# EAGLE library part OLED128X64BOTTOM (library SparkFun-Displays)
Micro OLED TODO: Add description SparkFun Products: product
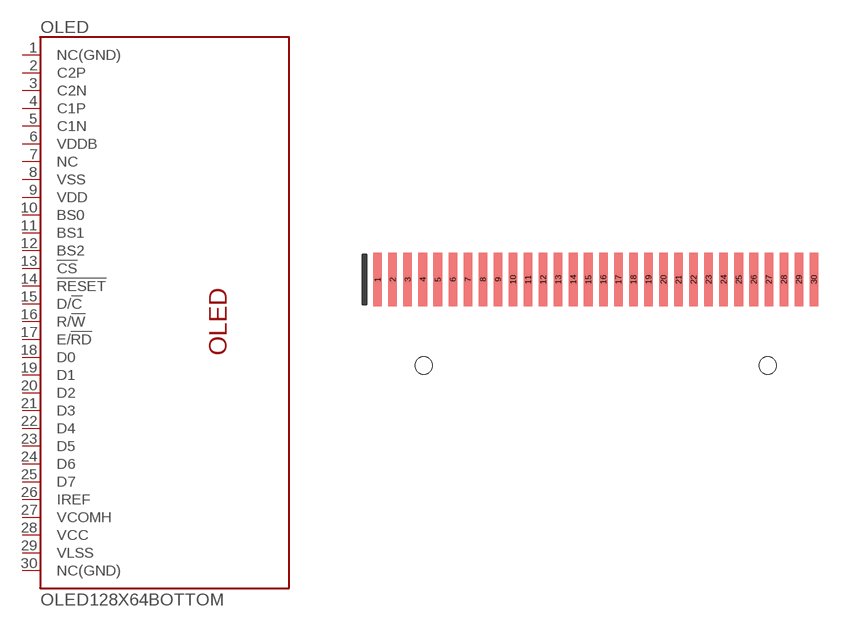
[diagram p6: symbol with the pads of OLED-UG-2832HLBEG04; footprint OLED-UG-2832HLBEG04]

Designator prefix OLED

## OLED128X64BOTTOM  [OLED-UG-2832HLBEG04]
1  NC(GND)
2  C2P
3  C2N
4  C1P
5  C1N
6  VDDB
7  NC
8  VSS
9  VDD
10  BS0
11  BS1
12  BS2
13  !CS!
14  !RESET!
15  D/!C!
16  R/!W!
17  E/!RD!
18  D0
19  D1
20  D2
21  D3
22  D4
23  D5
24  D6
25  D7
26  IREF
27  VCOMH
28  VCC
29  VLSS
30  NC(GND)

## Footprint OLED-UG-2832HLBEG04 (pad centres in mm)
OLDE display Specifications: Pin count: 30 Pin pitch: 0.7mm Area: Datasheet referenced for footprint: Example device(s): Microview breakout
smd 0.4 x 2.5: 1 0.85,-0.75; 2 1.55,-0.75; 3 2.25,-0.75; 4 2.95,-0.75; 5 3.65,-0.75; 6 4.35,-0.75; 7 5.05,-0.75; 8 5.75,-0.75; 9 6.45,-0.75; 10 7.15,-0.75; 11 7.85,-0.75; 12 8.55,-0.75; 13 9.25,-0.75; 14 9.95,-0.75; 15 10.65,-0.75; 16 11.35,-0.75; 17 12.05,-0.75; 18 12.75,-0.75; 19 13.45,-0.75; 20 14.15,-0.75; 21 14.85,-0.75; 22 15.55,-0.75; 23 16.25,-0.75; 24 16.95,-0.75; 25 17.65,-0.75; 26 18.35,-0.75; 27 19.05,-0.75; 28 19.75,-0.75; 29 20.45,-0.75; 30 21.15,-0.75
hole 0.8 at 19,-4.75
hole 0.8 at 3,-4.75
